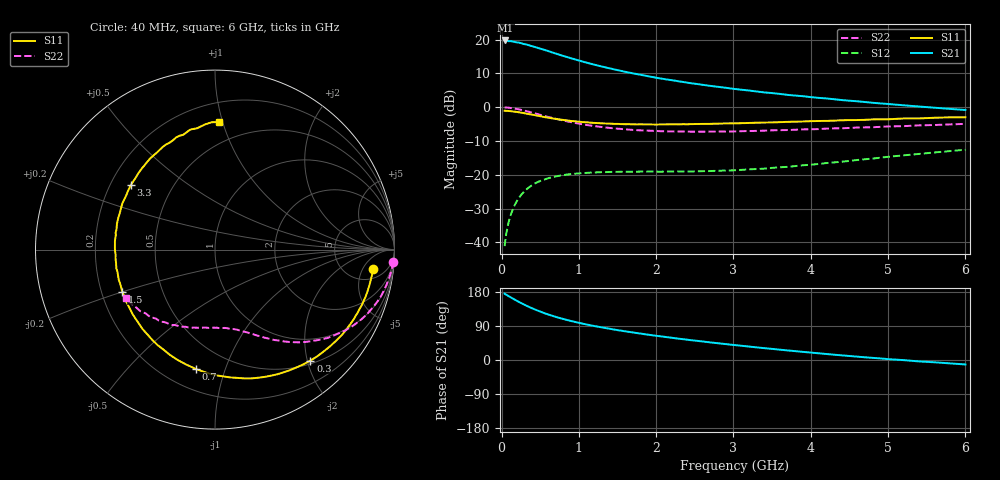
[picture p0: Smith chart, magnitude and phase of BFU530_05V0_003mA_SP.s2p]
! Filename:  P:\Prog\Test\Noise\ATS_data\Testdata_Net\03 Spar\BFU530_APG2013_40_A05_05p0V_003mA_SP_CM01_D.s2p
! Date/Time: Fri 26/Apr/2013 13:03:15
! BFU530_APG2013_40_A05_05p0V_1to25mA_SP_CM01_Bias3_R.s2p
! MDIF S-parameter v. bias file
! BFU530_APG2013_40_A05_05p0V_1to25mA_SP_CM01
! Date/time Wed Apr 24 19:36:53 2013
! VAR V_out= 5.0000
! VAR I_out= 2.9950
! VAR V_in= 0.8078
! VAR I_in= 0.0322
! Device data file deembeded for feedlines and parallel
! Original file: \03 Spar\BFU530_APG2013_40_A05_05p0V_003mA_SP_CM01_R.s2p
! Feed-files: PR047V01_250413_Feed1.s2p, PR047V01_250413_Feed2.s2p
! Parallel-file: PR047V01_250413_Par.s2p
# MHz S MA R 50
!  Freq-MHz  S11-mag  S11-arg  S21-mag  S21-arg  S12-mag  S12-arg  S22-mag  S22-arg
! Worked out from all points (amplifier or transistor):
!   98 points, 40 MHz to 6 GHz, reference 50 ohm
!   highest |S21| = 19.8 dB at 50 MHz (marker M1)
!   |S21| within 3 dB of that: start of sweep to 584.9 MHz
!   unconditionally stable (mu >= 1): 2.582 GHz to 4.615 GHz
!   at 300 MHz: K = 0.14, MSG = 21.7 dB, |S12| = -24.8 dB
!   at 1.6 GHz: K = 0.67, MSG = 14.8 dB, |S12| = -19.1 dB
!   at 6 GHz: K = 0.83, MSG = 5.9 dB, |S12| = -12.6 dB
!   S11 on the Smith chart (normalised r, x): 40 MHz: 8, -8; 300 MHz: 0.56, -2.05; 700 MHz: 0.33, -0.80; 1.5 GHz: 0.29, -0.20; 3.3 GHz: 0.28, +0.32; 6 GHz: 0.34, +0.97
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40  0.8886 -6.9  9.713 175.1  0.008825 85.7  0.9939 -3.9
50  0.8871 -8.6  9.725 173.1  0.0109 84.8  0.993 -4.9
70  0.8836 -11.9  9.613 171.5  0.01523 83.0  0.989 -6.9
120  0.8745 -20.6  9.508 165.2  0.02569 78.1  0.9752 -11.7
220  0.8444 -37.0  9.054 153.9  0.04475 68.9  0.9323 -20.8
300  0.8154 -49.3  8.577 145.5  0.05768 62.3  0.8892 -27.4
360  0.7905 -58.2  8.23 139.8  0.06602 57.9  0.8552 -31.7
460  0.7521 -71.8  7.61 131.1  0.0775 51.5  0.7975 -38.1
550  0.7173 -83.1  7.08 123.9  0.08504 46.5  0.7448 -43.1
700  0.6731 -99.2  6.237 113.9  0.0947 40.0  0.6752 -49.8
850  0.6385 -113.1  5.515 105.5  0.1012 35.1  0.6176 -55.1
1050  0.6038 -128.8  4.739 95.8  0.1061 30.3  0.5589 -61.1
1200  0.5869 -138.9  4.267 89.6  0.1085 27.7  0.5267 -64.7
1500  0.5674 -155.7  3.541 78.9  0.111 24.4  0.4827 -71.0
1750  0.5575 -167.5  3.092 71.1  0.1116 23.1  0.4587 -75.7
2050  0.5569 -179.1  2.673 62.7  0.1115 22.8  0.4431 -81.2
2450  0.5628 166.5  2.266 52.3  0.1122 23.9  0.4349 -88.6
3100  0.5812 147.5  1.817 37.6  0.1185 28.8  0.4425 -99.9
3300  0.591 142.3  1.711 33.3  0.1219 30.4  0.4474 -103.5
4100  0.6264 123.4  1.377 17.7  0.1449 35.3  0.4756 -117.9
5200  0.6829 101.6  1.069 -0.3  0.1944 35.1  0.5255 -137.5
6000  0.7107 88.2  0.911 -11.8  0.2354 30.5  0.5675 -151.5
